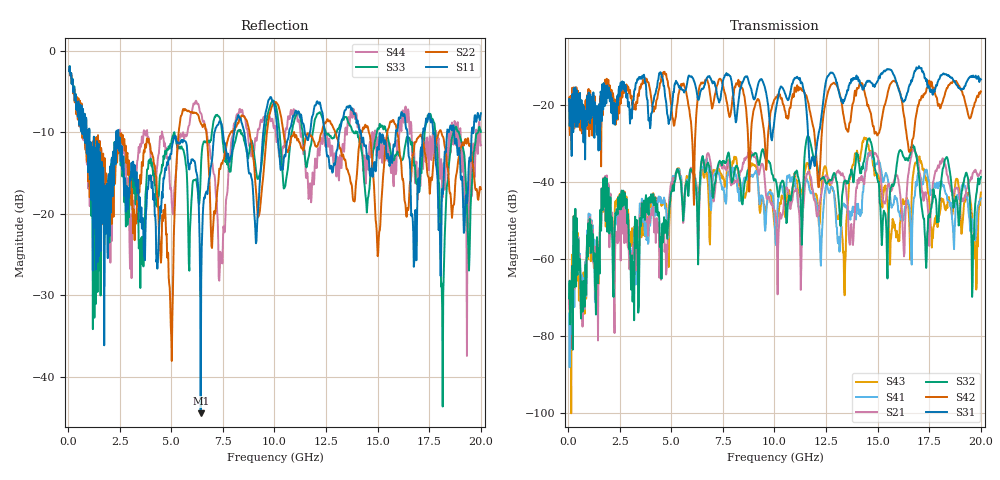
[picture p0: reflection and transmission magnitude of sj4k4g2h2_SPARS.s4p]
! FILE: E:\users\goganessyan\GBX_Backplane\FR408_backplane\1m_OUTBOUND_NEXT\sj4k4g2h2_SPARS.s4p
# MHZ S RI R 50.00
! FREQ  S11  S12  S13  S14
!  S21  S22  S23  S24
!  S31  S32  S33  S34
!  S41  S42  S43  S44
!  REAL  IMAG  REAL  IMAG  REAL  IMAG  REAL  IMAG
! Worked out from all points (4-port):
!   799 points, 50 MHz to 20 GHz, reference 50 ohm
!   strongest paths, dB at 50 MHz, 5.025 GHz, 10.03 GHz, 15.03 GHz, 20 GHz:
!     S31: -18.4, -20.2, -22.5, -13.5, -13.3
!     S42: -18.0, -21.8, -18.4, -27.4, -16.4
!     S32: -70.1, -42.2, -39.2, -40.0, -38.6
!     S21: -70.1, -40.2, -47.4, -33.8, -37.0
!     S41: -74.1, -39.7, -52.1, -34.4, -44.2
!     S43: -66.5, -41.7, -52.4, -38.2, -42.7
!   lowest |S11| = -44.5 dB at 6.425 GHz (marker M1), VSWR 1.01, Z = 49.4 + j0.116 ohm
!   |S11| at or under -10 dB: 1.027 GHz to 2.343 GHz (1.317 GHz wide, 78.1 % of centre); 2.43 GHz to 7.094 GHz (4.665 GHz wide, 98 % of centre); 14.18 GHz to 15.89 GHz (1.702 GHz wide, 11.3 % of centre)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
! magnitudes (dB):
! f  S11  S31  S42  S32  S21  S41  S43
! 50 MHz  -2.5  -18.4  -18.0  -70.1  -70.1  -74.1  -66.5
! 1.725 GHz  -17.6  -14.3  -14.4  -39.5  -39.5  -39.8  -39.7
! 5 GHz  -12.7  -21.3  -20.1  -42.6  -40.2  -40.0  -42.1
! 6.425 GHz  -44.5  -16.3  -14.5  -36.4  -37.3  -39.0  -37.8
! 12.12 GHz  -6.5  -27.8  -41.3  -37.6  -48.1  -47.9  -47.8
! 12.82 GHz  -14.9  -11.7  -14.4  -38.3  -39.5  -41.5  -42.0
! 20 GHz  -7.7  -13.3  -16.4  -38.6  -37.0  -44.2  -42.7
